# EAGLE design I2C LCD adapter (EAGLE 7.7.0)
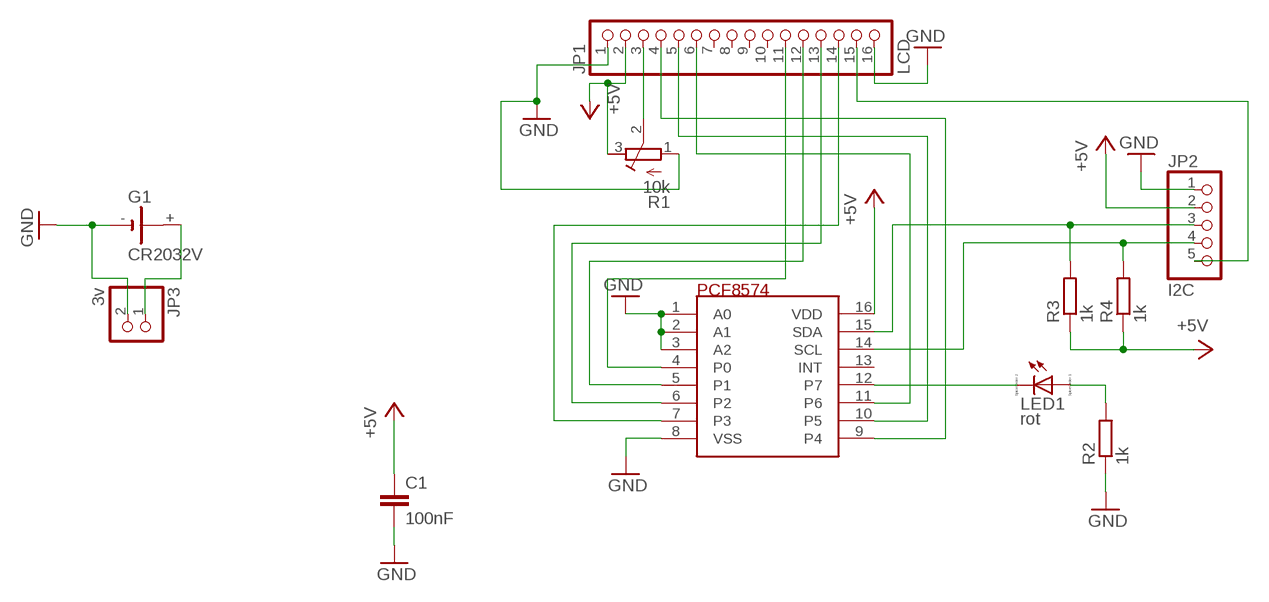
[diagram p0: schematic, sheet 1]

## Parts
C1  100nF  C-EUC1206  [C1206]
G1  CR2032V  [CR2032V]
JP1  LCD  PINHD-1X16  [1X16]
JP2  I2C  PINHD-1X5  [1X05]
JP3  3v  PINHD-1X2  [1X02]
LED1  rot  LED_E  [LED_1206]
R1  10k  R-TRIMM64W  [RTRIM64W]
R2  1k  R-EU_M1206  [M1206]
R3  1k  R-EU_M1206  [M1206]
R4  1k  R-EU_M1206  [M1206]
U$1  PCF8574  [SOP16_9.53MM]

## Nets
+5V: C1.1 JP1.2 JP2.2 R1.3(E) R3.1 R4.1 U$1.16(VDD)
GND: C1.2 G1.- JP1.1 JP1.16 JP2.1 JP3.2 R1.1(A) R2.1 U$1.1(A0) U$1.2(A1) U$1.3(A2) U$1.8(VSS)
LED: LED1.C U$1.12(P7)
N$2: G1.+ JP3.1
N$3: JP1.6 U$1.11(P6)
N$4: JP1.5 U$1.10(P5)
N$5: JP1.4 U$1.9(P4)
N$6: JP1.3 R1.2(S)
N$8: JP1.11 U$1.4(P0)
N$9: JP1.12 U$1.5(P1)
N$10: JP1.13 U$1.6(P2)
N$11: JP1.14 U$1.7(P3)
N$13: JP1.15 JP2.5
N$14: LED1.A R2.2
SCL: JP2.4 R4.2 U$1.14(SCL)
SDA: JP2.3 R3.2 U$1.15(SDA)
Unconnected: G1.+@1(+) JP1.7 JP1.8 JP1.9 JP1.10 U$1.13(INT)

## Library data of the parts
C1 = resistor:C-EU: CAPACITOR, European symbol
G1 = battery:CR2032V: LI BATTERY Varta
JP1 = pinhead:PINHD-1X16: PIN HEADER
JP2 = pinhead:PINHD-1X5: PIN HEADER
JP3 = pinhead:PINHD-1X2: PIN HEADER
LED1 = eagle-ltspice:LED_E: LED; SPICEMODEL: NONE; SPICEPREFIX: D; SPICETYPE: diode
R1 = resistor:R-TRIMM: Trimm resistor
R2-R4 = resistor:R-EU_: RESISTOR, European symbol
U$1 = PCF8574:PCF8574

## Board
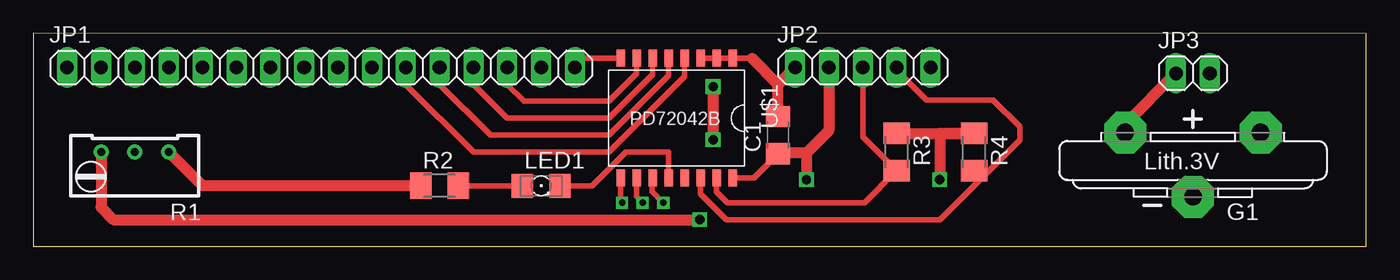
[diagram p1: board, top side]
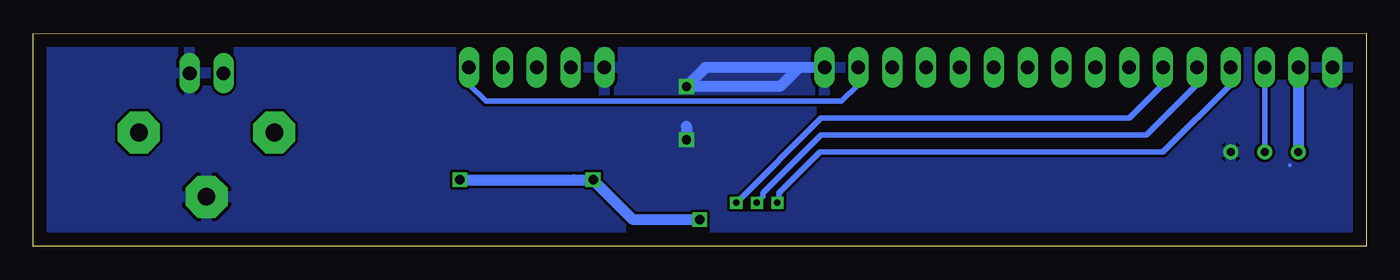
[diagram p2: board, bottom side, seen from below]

Size 100 x 16 mm. Coordinates in mm from the lower left corner, seen from the top.
Outline: 0,0 100,0 100,15.96 0,16 0,0
Copper layers (1*16): Top 0.035mm / dielectric 1.5mm / Bottom 0.035mm
Design rules "default": minimum track width 10mil, minimum drill 24mil, track to track 8mil, track to pad 8mil, pad to pad 8mil, via to via 8mil, smd to smd 8mil, copper to edge 40mil, drill to drill 8mil, minimum pad ring 10mil, minimum via ring 8mil, stop-mask expansion 4mil, vias tented up to drill 0mil, thermal gap 10mil

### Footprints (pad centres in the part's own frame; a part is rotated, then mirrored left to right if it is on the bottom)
C1206 = smd 1.6 x 1.8: 1 -1.4,0; 2 1.4,0
CR2032V = drill 1.321 pad 3.15 octagon: + -2.54,-5.08; +@1 -2.54,5.08; - 2.286,0
1X16 = drill 1.016 long: 1 -19.05,0; 2 -16.51,0; 3 -13.97,0; 4 -11.43,0; 5 -8.89,0; 6 -6.35,0; 7 -3.81,0; 8 -1.27,0; 9 1.27,0; 10 3.81,0; 11 6.35,0; 12 8.89,0; 13 11.43,0; 14 13.97,0; 15 16.51,0; 16 19.05,0
1X05 = drill 1.016 long: 1 -5.08,0; 2 -2.54,0; 3 0,0; 4 2.54,0; 5 5.08,0
1X02 = drill 1.016 long: 1 -1.27,0; 2 1.27,0
LED_1206 = smd 1.6 x 1.803: A -1.422,0; C 1.422,0
RTRIM64W = drill 0.61: 1 1.27,-2.54; 2 1.27,0; 3 1.27,2.54
M1206 = smd 1.6 x 2: 1 -1.4,0; 2 1.4,0
SOP16_9.53MM = smd 0.635 x 1.27: 1 -4.2,-4.5; 2 -3,-4.5; 3 -1.8,-4.5; 4 -0.6,-4.5; 5 0.6,-4.5; 6 1.8,-4.5; 7 3,-4.5; 8 4.2,-4.5; 9 4.2,4.5; 10 3,4.5; 11 1.8,4.5; 12 0.6,4.5; 13 -0.6,4.5; 14 -1.8,4.5; 15 -3,4.5; 16 -4.2,4.5

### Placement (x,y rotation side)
C1  55.88,8.35 90 top
G1  87,6 270 top
JP1  21.59,13.43 0 top
JP2  62.23,13.43 0 top
JP3  87,13 0 top
LED1  38.1,4.54 0 top
R1  7.62,5.81 90 top
R2  30.48,4.54 0 top
R3  64.77,7.08 270 top
R4  70.58,7.08 270 top
U$1  48.26,9.62 180 top

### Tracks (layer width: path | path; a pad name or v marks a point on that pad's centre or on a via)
+5V  (via drill 0.7)  (1 unrouted)
  Top 0.406: U$1.16 54.05,5.12 C1.1
  Top 0.813: 68,8.48 R4.1 R3.1 68,8.48 | 68,8.48 v68,5 | JP2.2 59.69,8.69 58,7 | 58,7 55.93,7 C1.1 | 58,7 58,5 | R1.3 5.08,2.92 6,2 v50,2
  Bottom 0.254: 59.44,5.2 59.44,5
  Bottom 0.813: v68,5 59.44,5 58,5 55,2 v50,2 | JP1.2 R1.3
GND  (via drill 0.7)
  Top 0.406: 53.92,14.12 U$1.1 U$1.2 U$1.3 | U$1.8 41.33,14.12 JP1.16
  Top 0.813: C1.2 55.88,12.16 | 55.88,12.16 JP2.1 | 53.92,14.12 55.88,12.16 | R1.1 12.7,4.54 R2.1 24.54,4.54 | v51,12 v51,8
  Bottom 0.254: 5.71,6.12 5.73,6.08
  Bottom 0.813: 51,9 v51,8 | JP1.16 42.57,13.43 44,12 v51,12 49.57,13.43 JP1.16
  pour Bottom: 0,0 0,16 100,16 100,0
LED
  Top 0.406: LED1.C 41.91,4.54 44.45,7.08 47.66,7.08 U$1.12
N$1  (via drill 0.7)
  other vias: 58,5
N$2
  Top 0.813: G1.+ 81.92,9.19 JP3.1
N$3  (via drill 0.5)
  Top 0.406: U$1.11 46.46,4.83 46.42,4.87 46.42,4.11 v47.26,3.27
  Bottom 0.406: JP1.6 15.24,12.16 17.78,9.62 40.91,9.62 v47.26,3.27
N$4  (via drill 0.5)
  Top 0.406: U$1.10 45.26,3.73 v45.72,3.27
  Bottom 0.406: JP1.5 12.7,12.16 16.51,8.35 40.91,8.35 45.26,4 45.26,3.73 v45.72,3.27
N$5  (via drill 0.5)
  Top 0.406: U$1.9 44.06,3.39 v44.18,3.27
  Bottom 0.406: JP1.4 10.16,12.16 15.24,7.08 40.98,7.08 44.06,4 44.06,3.39 v44.18,3.27
N$6
  Bottom 0.406: JP1.3 R1.2
N$8
  Top 0.406: U$1.4 48.86,12.76 43.18,7.08 33.02,7.08 27.94,12.16 JP1.11
N$9
  Top 0.406: U$1.5 47.66,12.83 43.18,8.35 34.29,8.35 30.48,12.16 JP1.12
N$10
  Top 0.406: U$1.6 46.46,12.9 43.18,9.62 35.56,9.62 33.02,12.16 JP1.13
N$11
  Top 0.406: U$1.7 45.26,12.97 43.18,10.89 36.83,10.89 35.56,12.16 JP1.14
N$13
  Bottom 0.406: JP1.15 38.1,12.16 39.37,10.89 66.04,10.89 67.31,12.16 JP2.5
N$14
  Top 0.406: LED1.A R2.2
SCL
  Top 0.406: U$1.14 50.06,3.94 52,2 68,2 71,5 | JP2.4 64.77,13.23 67,11 72,11 74,9 74,8 71,5 | 71,5 71,5.26 R4.2
SDA
  Top 0.406: JP2.3 62.23,8.22 R3.2 62.36,3.27 52.07,3.27 51.26,4.08 U$1.15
